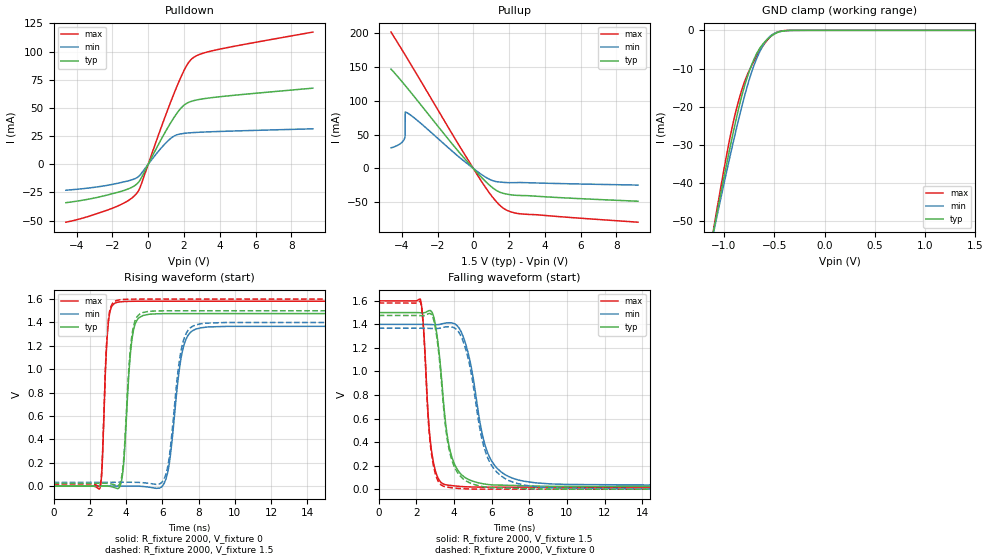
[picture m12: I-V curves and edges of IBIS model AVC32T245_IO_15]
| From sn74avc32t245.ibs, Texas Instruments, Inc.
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[Model]   AVC32T245_IO_15
Model_type  I/O
Vinl=0.49
Vinh=1.04
Enable   Active-Low
Vref =   0
Rref =   2000
Cref =   15p
Vmeas =   0.75
| variable   typ   min   max
C_comp   5.18pF   4.55pF   5.77pF
| C_pullup   5.10pF   3.65pF   7.53pF
| C_pulldown   4.79pF   4.27pF   5.46pF
| C_tri-state   5.18pF   4.55pF   5.77pF
[Temperature Range]   40   100   -40
| Ambient temperature   25   85   -40
[Voltage range]   1.5   1.4   1.6
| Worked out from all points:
|   slope of the pulldown table from 0 to 0.225 V, typ, clamps not added: 32.1 ohm
|   slope of the pullup table from 0 to 0.225 V, typ, clamps not added: 33.9 ohm
|   GND clamp passes 1 mA (typ) near -0.50 V on its own axis
|   rising waveform, R_fixture 2000, V_fixture 0: 20-80 % time 355ps typ, 581ps min, 236ps max; typ from 0 V to 1.48 V
|   falling waveform, R_fixture 2000, V_fixture 1.5: 20-80 % time 628ps typ, 1ns min, 383ps max; typ from 1.5 V to 0.023 V
|   rising waveform, R_fixture 2000, V_fixture 1.5: 20-80 % time 351ps typ, 568ps min, 235ps max; typ from 0.023 V to 1.5 V
|   falling waveform, R_fixture 2000, V_fixture 0: 20-80 % time 629ps typ, 997ps min, 376ps max; typ from 1.48 V to 0 V
[GND Clamp]
| AVC32T245_IO_15
|   Voltage   I(typ)   I(min)   I(max)
-4.6V     -597.8mA   -546.6mA   -662.5mA
-1.1V     -52.11mA   -52.52mA   -51.59mA
-1.075V   -48.66mA   -49.4mA    -47.7mA
-930mV    -29.5mA    -31.88mA   -26.82mA
-830mV    -17.94mA   -20.74mA   -16.24mA
-765mV    -12.02mA   -14.35mA   -11.48mA
-685mV    -6.644mA   -8.056mA   -7.261mA
-605mV    -3.35mA    -3.664mA   -3.806mA
-535mV    -1.602mA   -1.422mA   -1.608mA
-460mV    -500.6uA   -413.1uA   -383.6uA
-350mV    -38.76uA   -40.58uA   -15.38uA
1.5V      804.6pA    34.44nA    79.67pA
[Pulldown]
| AVC32T245_IO_15
|   Voltage   I(typ)   I(min)   I(max)
-4.6V     -34.07mA   -23.01mA   -51.35mA
-1.885V   -25.62mA   -17.44mA   -38.24mA
-1.09V    -21.68mA   -14.59mA   -31.97mA
-630mV    -17.39mA   -11.88mA   -25.55mA
-415mV    -12.94mA   -8.777mA   -18.95mA
595mV     18.22mA    11.97mA    26.91mA
1.265V    37.01mA    23.01mA    55.56mA
1.7V      47.29mA    26.56mA    72.61mA
2.03V     52.78mA    27.45mA    84.03mA
2.5V      56.24mA    28.09mA    94.31mA
3.84V     59.63mA    29.04mA    101.6mA
9.2V      67.51mA    31.46mA    117.2mA
[Pullup]
| AVC32T245_IO_15
|   Voltage   I(typ)   I(min)   I(max)
-4.6V     146.8mA    30.47mA    201.5mA
-4.1V     131.8mA    36.24mA    180.2mA
-3.85V    123.9mA    43.96mA    169.4mA
-3.81V    122.6mA    49.37mA    167.6mA
-3.805V   122.5mA    83.3mA     167.4mA
-3.785V   121.8mA    83.17mA    166.5mA
-3.155V   101.3mA    71.56mA    138.8mA
175mV     -5.197mA   -3.574mA   -7.497mA
980mV     -26.35mA   -16.94mA   -39.04mA
1.625V    -36.35mA   -20.39mA   -57.65mA
2.595V    -39.89mA   -20.78mA   -66.9mA
9.2V      -48.41mA   -24.54mA   -79.36mA
[Ramp]
| AVC32T245_IO_15
| variable   typ   min   max
dV/dt_r   0.90/3.68E-10   0.83/5.92E-10   0.96/2.50E-10
dV/dt_f   0.90/6.38E-10   0.83/1.01E-09   0.96/3.92E-10
R_load = 2000
[Rising Waveform]
| AVC32T245_IO_15
R_fixture =   2000
C_fixture =   0
L_fixture =   0
V_fixture =   0
V_fixture_min = 0
V_fixture_max = 0
|   Time   V(typ)   V(min)   V(max)
0s        19.4nV     97.73nV    508.8pV
2.565ns   916.4uV    -148.7uV   -15.7mV
2.99ns    18.64uV    135.2uV    1.342V
3.425ns   -16.85mV   571uV      1.568V
4.36ns    1.291V     546.3uV    1.581V
4.925ns   1.459V     -2.673mV   1.582V
6.19ns    1.475V     56.84mV    1.582V
7.08ns    1.475V     1.134V     1.582V
7.865ns   1.475V     1.344V     1.582V
29.99ns   1.476V     1.367V     1.582V
[Falling Waveform]
| AVC32T245_IO_15
R_fixture =   2000
C_fixture =   0
L_fixture =   0
V_fixture =   1.5
V_fixture_min = 1.4
V_fixture_max = 1.6
|   Time   V(typ)   V(min)   V(max)
0s        1.5V       1.4V       1.6V
2.21ns    1.499V     1.4V       1.615V
2.795ns   1.511V     1.398V     340.3mV
3.115ns   1.288V     1.398V     108.7mV
3.475ns   685.3mV    1.409V     41.69mV
3.805ns   319.6mV    1.413V     31.82mV
4.35ns    131.5mV    1.347V     22.95mV
5.74ns    40.93mV    330.2mV    17.41mV
7.215ns   31.29mV    87.56mV    17.21mV
29.99ns   23.49mV    32.46mV    17.19mV
[Rising Waveform]
| AVC32T245_IO_15
R_fixture =   2000
C_fixture =   0
L_fixture =   0
V_fixture =   1.5
V_fixture_min = 1.4
V_fixture_max = 1.6
|   Time   V(typ)   V(min)   V(max)
0s        23.49mV    32.45mV    17.19mV
2.56ns    24.39mV    32.33mV    -123.6uV
3ns       23.29mV    32.62mV    1.385V
3.485ns   3.982mV    33.1mV     1.588V
4.33ns    1.297V     32.85mV    1.599V
4.91ns    1.484V     29.77mV    1.6V
6.175ns   1.5V       91.38mV    1.6V
7.04ns    1.5V       1.165V     1.6V
7.81ns    1.5V       1.377V     1.6V
29.99ns   1.5V       1.4V       1.6V
[Falling Waveform]
| AVC32T245_IO_15
R_fixture =   2000
C_fixture =   0
L_fixture =   0
V_fixture =   0
V_fixture_min = 0
V_fixture_max = 0
|   Time   V(typ)   V(min)   V(max)
0s        1.476V     1.367V     1.582V
2.21ns    1.474V     1.367V     1.596V
2.79ns    1.486V     1.365V     320.3mV
3.105ns   1.271V     1.365V     87.05mV
3.455ns   682.8mV    1.375V     24.36mV
3.79ns    303.1mV    1.379V     14.05mV
4.325ns   112.7mV    1.315V     5.375mV
5.715ns   16.97mV    296.9mV    209.3uV
7.21ns    7.308mV    54.89mV    22uV
29.99ns   175.2nV    3.764uV    32.44nV
